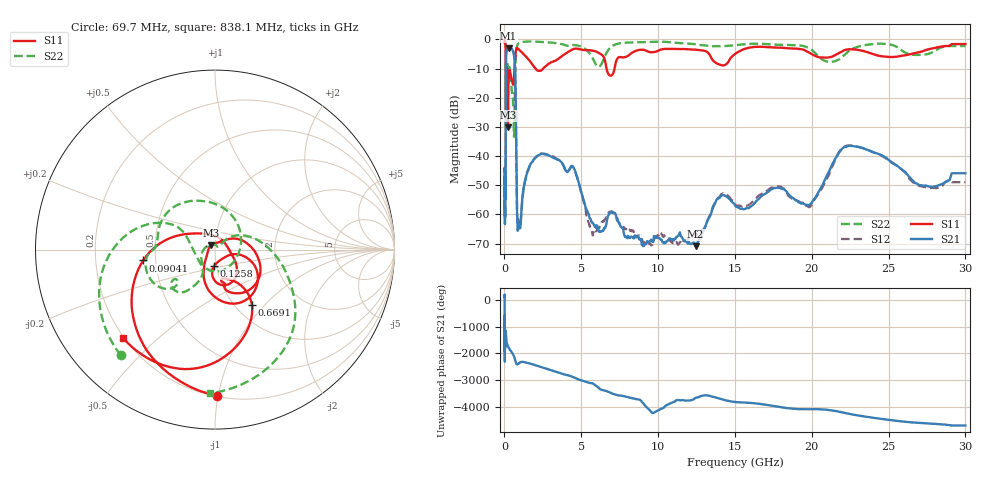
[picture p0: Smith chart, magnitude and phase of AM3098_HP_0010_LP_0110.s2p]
! Date/Time: Thu, Feb 28, 2019 8:33 AM
! Network Analyzer: Agilent Technologies E8364B Rev: A.07.50.67
! Sweep from 0.010 to 30.000 GHz, 1601 Points, Sweep Type: LOG
! Power Supply: 5.023 V, 0.002 A
# Hz S DB R 50
!freq MagS11 AngS11 MagS21 AngS21 MagS12 AngS12 MagS22 AngS22
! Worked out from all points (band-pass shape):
!   1601 points, 10 MHz to 30 GHz, reference 50 ohm
!   highest |S21| = -3.09 dB at 266.5 MHz (marker M1); lowest = -70.9 dB at 12.43 GHz (marker M2)
!   |S21| within 3 dB of the highest: 106.1 MHz to 640.7 MHz (534.6 MHz wide, 143 % of centre)
!   lowest |S11| = -30.1 dB at 227 MHz (marker M3), VSWR 1.06, Z = 47.9 + j2.24 ohm
!   |S11| at or under -10 dB: 176 MHz to 655.6 MHz (479.6 MHz wide, 115 % of centre); 2.028 GHz to 2.521 GHz (492.2 MHz wide, 21.6 % of centre); 6.643 GHz to 7.166 GHz (522.7 MHz wide, 7.57 % of centre)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
!   |S22| runs from -33.4 to -0.5 dB; largest |S21 - S12| = 0.012
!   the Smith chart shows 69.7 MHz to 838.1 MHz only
!   S11 on the Smith chart (normalised r, x): 69.7 MHz: 0.21, -0.99; 90.41 MHz: 0.43, -0.06; 125.8 MHz: 0.97, -0.18; 669.1 MHz: 1.19, -0.84; 838.1 MHz: 0.20, -0.39
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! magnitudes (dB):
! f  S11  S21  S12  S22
! 10 MHz  -0.4  -45.0  -45.2  -0.5
! 38.04 MHz  -0.5  -60.1  -60.3  -0.9
! 69.7 MHz  -1.8  -53.0  -52.8  -2.1
! 90.41 MHz  -7.9  -19.6  -19.6  -9.3
! 125.8 MHz  -20.8  -4.3  -4.3  -10.7
! 144.7 MHz  -13.7  -3.7  -3.6  -10.3
! 185.8 MHz  -11.3  -3.5  -3.5  -8.1
! 227 MHz  -30.1  -3.2  -3.1  -9.5
! 266.5 MHz  -14.5  -3.1  -3.0  -9.7
! 550.5 MHz  -15.5  -3.9  -3.9  -20.4
! 620.7 MHz  -13.1  -5.3  -5.2  -33.3
! 669.1 MHz  -8.7  -8.0  -8.0  -20.8
! 838.1 MHz  -3.0  -63.3  -62.4  -1.9
! 2.084 GHz  -10.4  -40.2  -40.2  -0.8
! 4.458 GHz  -3.3  -43.5  -43.7  -2.0
! 5.668 GHz  -3.8  -62.7  -65.2  -5.8
! 7.926 GHz  -5.9  -67.6  -65.1  -1.1
! 12.43 GHz  -3.5  -70.9  -67.1  -1.6
! 14.09 GHz  -8.8  -53.6  -53.1  -2.3
! 19.8 GHz  -4.5  -56.9  -57.5  -2.9
! 22.56 GHz  -3.4  -36.5  -36.3  -3.5
! 30 GHz  -1.6  -45.9  -48.9  -2.3
